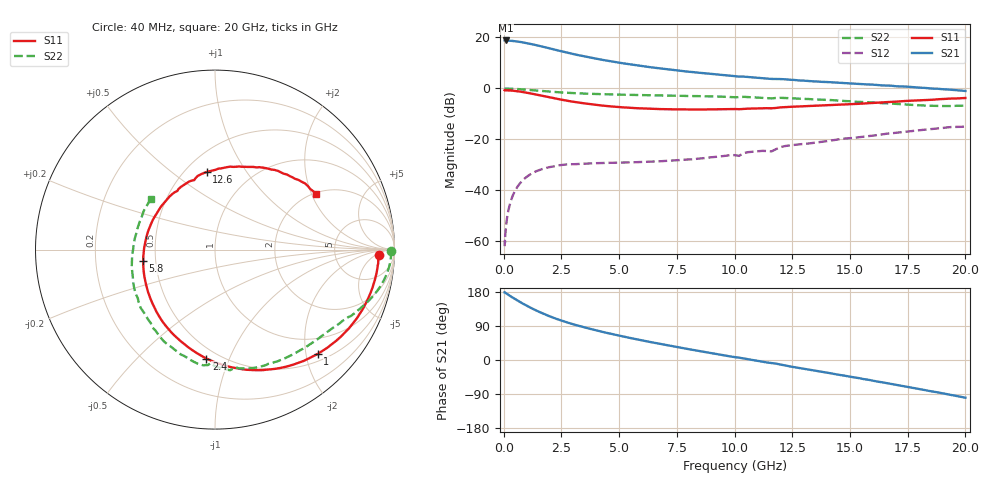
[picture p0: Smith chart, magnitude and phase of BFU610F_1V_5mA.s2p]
! Filename:  P:\Prog\Test\Noise\ATS_data\Testdata_Net\SplitFiles\BFU610_2W_A5_HighFreq_1V_5mA_D.s2p
! Date/Time: Wed 10/Aug/2011 16:54:47
! BFU610_2W_A5_HighFreq_1V_1mA_10mA_Bias4_R.s2p
! MDIF S-parameter v. bias file
! BFU610_2W_A5_HighFreq_1V_1mA_10mA
! Date/time Mon Aug 08 13:53:02 2011
! VAR V_out= 1.0000
! VAR I_out= 4.9950
! VAR V_in= 0.9086
! VAR I_in= 0.0419
! Device data file deembeded for feedlines and parallel
! Original file: \SplitFiles\BFU610_2W_A5_HighFreq_1V_5mA_R.s2p
! Feed-files: PR003V01_101208_Feed1.s2p, PR003V01_101208_Feed2.s2p
! Parallel-file: PR003V01_101208_Par.s2p
# MHz S MA R 50
!  Freq-MHz  S11-mag  S11-arg  S21-mag  S21-arg  S12-mag  S12-arg  S22-mag  S22-arg
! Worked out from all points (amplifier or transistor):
!   167 points, 40 MHz to 20 GHz, reference 50 ohm
!   highest |S21| = 18.7 dB at 80 MHz (marker M1)
!   |S21| within 3 dB of that: start of sweep to 1.945 GHz
!   unconditionally stable (mu >= 1): 3.279 GHz to end of sweep
!   at 550 MHz: K = 0.15, MSG = 28.8 dB, |S12| = -39.3 dB
!   at 4.2 GHz: K = 1.31, MAG = 17.0 dB, |S12| = -29.3 dB
!   at 20 GHz: K = 1.45, MAG = 3.0 dB, |S12| = -15.0 dB
!   S11 on the Smith chart (normalised r, x): 40 MHz: 19, -7; 1 GHz: 0.64, -2.24; 2.4 GHz: 0.43, -0.83; 5.8 GHz: 0.43, -0.07; 12.6 GHz: 0.63, +0.68; 20 GHz: 2.05, +2.16
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40  0.9127 -1.9  8.62 178.6  0.0008037 87.3  0.9803 -0.4
80  0.9116 -3.8  8.621 176.9  0.001542 87.2  0.9818 -1.1
140  0.9107 -6.7  8.583 174.5  0.002753 87.0  0.9814 -2.0
260  0.9046 -12.4  8.539 169.8  0.005188 84.5  0.979 -3.9
600  0.8715 -28.2  8.22 156.8  0.01179 74.3  0.963 -8.9
800  0.8451 -36.9  7.938 149.8  0.01529 68.7  0.9494 -11.6
1000  0.8158 -45.4  7.627 143.2  0.01845 63.5  0.9339 -14.1
1300  0.769 -57.3  7.156 133.8  0.02235 56.7  0.9099 -17.4
1650  0.7142 -70.2  6.573 124.0  0.0259 49.9  0.8825 -20.9
2100  0.6473 -85.3  5.859 112.7  0.02904 42.9  0.8518 -24.8
2400  0.609 -94.5  5.426 106.2  0.03093 39.2  0.8303 -27.1
2900  0.5532 -108.2  4.805 96.3  0.03235 33.4  0.8075 -30.5
3400  0.5115 -120.8  4.289 87.7  0.03307 30.7  0.7874 -33.9
4400  0.4505 -143.4  3.513 72.5  0.03431 27.1  0.7613 -40.4
5800  0.4052 -170.7  2.792 54.1  0.03562 26.7  0.7357 -49.7
6800  0.3896 172.0  2.431 42.2  0.03711 28.2  0.7211 -56.6
8800  0.3848 141.4  1.941 20.0  0.0432 33.1  0.6957 -70.9
10200  0.3881 122.7  1.689 6.1  0.04729 36.6  0.6675 -80.4
12600  0.4351 96.1  1.45 -19.0  0.07752 32.8  0.6301 -102.5
13400  0.4513 87.6  1.364 -27.1  0.08471 29.0  0.6054 -110.5
16800  0.5403 56.5  1.118 -63.4  0.131 8.9  0.4989 -154.4
20000  0.6433 28.8  0.8833 -99.5  0.1774 -21.8  0.4545 142.0
